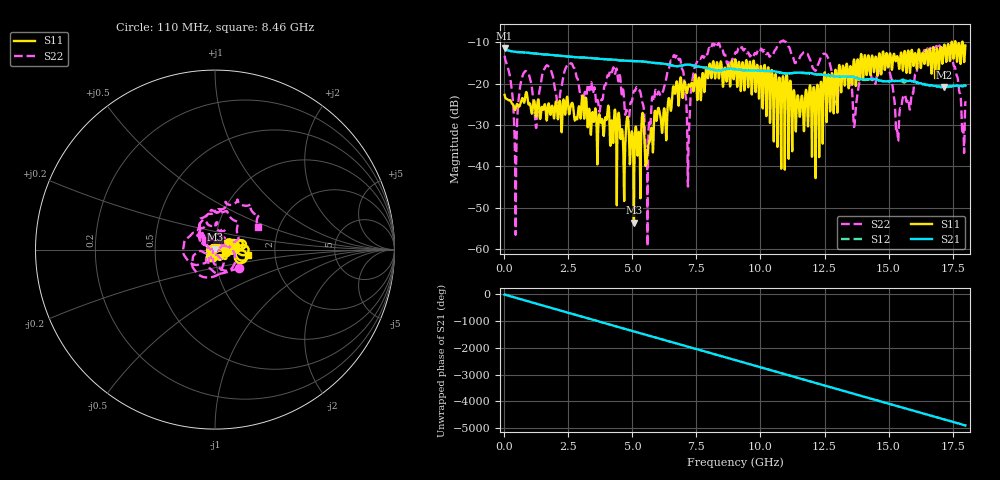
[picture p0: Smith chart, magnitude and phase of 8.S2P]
!Agilent Technologies,E5071C,MY46316741,A.11.02
!Date: Thu Sep 29 15:31:22 2022
!Data & Calibration Information:
!Freq	S11:SOLT2(ON)	S21:SOLT2(ON)	S12:SOLT2(ON)	S22:SOLT2(ON)
!PortZ  Port1:50+j0  Port2:50+j0
!Above PortZ is port z conversion or system Z0 setting when saving the data.
!When reading, reference impedance value at option line is always used.
# Hz S dB R 50
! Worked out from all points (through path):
!   1800 points, 10 MHz to 18 GHz, reference 50 ohm
!   highest |S21| = -11.35 dB at 10 MHz (marker M1); lowest = -20.8 dB at 17.18 GHz (marker M2)
!   group delay of S21, straight-line fit = 756 ps
!   lowest |S11| = -53.6 dB at 5.06 GHz (marker M3), VSWR 1.00, Z = 50 + j0.208 ohm
!   |S11| at or under -10 dB: start of sweep to 17.46 GHz; 17.48 GHz to 17.59 GHz (110.1 MHz wide, 0.628 % of centre); 17.62 GHz to 17.87 GHz (251.8 MHz wide, 1.42 % of centre)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
!   |S22| runs from -59.3 to -9.5 dB; largest |S21 - S12| = 0.011
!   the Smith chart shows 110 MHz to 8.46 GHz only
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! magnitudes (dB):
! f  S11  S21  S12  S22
! 10 MHz  -22.7  -11.3  -11.4  -13.2
! 440 MHz  -26.0  -12.3  -12.3  -56.6
! 810 MHz  -23.4  -12.4  -12.4  -17.0
! 1.23 GHz  -27.8  -12.7  -12.7  -30.5
! 1.66 GHz  -28.8  -12.9  -12.9  -15.5
! 3.01 GHz  -25.2  -13.6  -13.6  -22.3
! 5.06 GHz  -53.6  -14.5  -14.5  -21.7
! 5.57 GHz  -37.7  -14.7  -14.7  -38.3
! 6.01 GHz  -25.8  -15.0  -15.0  -22.0
! 6.8 GHz  -25.3  -15.7  -15.7  -14.1
! 7.18 GHz  -20.5  -15.4  -15.4  -38.2
! 7.53 GHz  -23.9  -15.8  -15.8  -14.6
! 9.01 GHz  -14.3  -16.5  -16.5  -12.6
! 12.01 GHz  -37.7  -17.5  -17.5  -15.6
! 13.36 GHz  -15.2  -18.3  -18.3  -17.0
! 13.68 GHz  -15.3  -18.5  -18.4  -29.4
! 14.03 GHz  -16.3  -18.9  -19.1  -16.1
! 15.01 GHz  -15.0  -19.4  -19.4  -16.4
! 15.35 GHz  -13.4  -19.3  -19.3  -31.9
! 16.33 GHz  -12.5  -20.1  -20.2  -13.4
! 17.18 GHz  -10.5  -20.8  -20.9  -12.0
! 18 GHz  -10.7  -20.5  -20.6  -24.2
